{attribute 'qualified_only'}
VAR_GLOBAL
//************************HW-IO******************************************
	NDI:STR_NDI;	
	NDO:STR_NDO;
	AI:STR_AI;
	AO:STR_AO;
	
	//POWER
	TURBO_PUMP_POWER_ON :BOOL;
	PENDULUM_VALVE_HEATER_POWER_ON:BOOL;
	LID_HEATER_POWER_ON:BOOL;
	CHAMBER_HEATER_POWER_ON:BOOL;
	IGS_HEATER_POWER_ON:BOOL;
	TAPE_HEATER_POWER_ON:BOOL;
	FORELINE_HEATER_POWER_ON:BOOL;
	GATE_VALVE_HEATER_POWER_ON:BOOL;
	
	//HEATER	
	LID_HEATER_AUTO_TUNE_EN				:ARRAY[1..10] OF BOOL;
	CHAMBER_HEATER_AUTO_TUNE_EN			:ARRAY[1..10] OF BOOL;
	PEN_VALVE_HEATER_AUTO_TUNE_EN		:BOOL;
	GATE_VALVE_HEATER_AUTO_TUNE_EN		:BOOL;
	IGS_HEATER_AUTO_TUNE_EN				:ARRAY[1..10] OF BOOL;
	TAPE_HEATER_AUTO_TUNE_EN			:ARRAY[1..10] OF BOOL;
	FORELINE_HEATER_AUTO_TUNE_EN		:ARRAY[1..20] OF BOOL;
	STAGE_HEATER_AUTO_TUNE_EN			:ARRAY[1..10] OF BOOL;
	
	LID_HEATER_AUTO_TUNE_OUTPUT			:ARRAY[1..10] OF REAL;
	CHAMBER_HEATER_AUTO_TUNE_OUTPUT		:ARRAY[1..10] OF REAL;
	PEN_VALVE_HEATER_AUTO_TUNE_OUTPUT	:REAL;
	GATE_VALVE_HEATER_AUTO_TUNE_OUTPUT	:REAL;
	IGS_HEATER_AUTO_TUNE_OUTPUT			:ARRAY[1..10] OF REAL;
	TAPE_HEATER_AUTO_TUNE_OUTPUT		:ARRAY[1..10] OF REAL;
	FORELINE_HEATER_AUTO_TUNE_OUTPUT	:ARRAY[1..20] OF REAL;
	STAGE_HEATER_AUTO_TUNE_OUTPUT		:ARRAY[1..10] OF REAL;
	
	LID_HEATER_SSR_ON					:ARRAY[1..10] OF BOOL;
	CHAMBER_HEATER_SSR_ON				:ARRAY[1..10] OF BOOL;
	PEN_VALVE_HEATER_SSR_ON				:BOOL;
	GATE_VALVE_SSR_ON					:BOOL;
	IGS_HEATER_SSR_ON					:ARRAY[1..10] OF BOOL;
	TAPE_HEATER_SSR_ON					:ARRAY[1..10] OF BOOL;
	FORELINE_HEATER_SSR_ON				:ARRAY[1..20] OF BOOL;
	STAGE_HEATER_SCR_OUTPUT				:ARRAY[1..10] OF REAL;
	
//INTERLOCK
	ALARM_OCC:BOOL;
	WARNING_OCC:BOOL;
	
//UI-Config
	PMConfig:ConfigPM;
	
	MFCVerification:ConfigMfcVer;
	
	Chiller:ConfigChiller;	
	InnerChiller:ConfigChiller;
	OuterChiller:ConfigChiller;
	TopChiller:ConfigChiller;
	
	DryPump:ConfigDryPump;
	
	Mfcgas1					:ConfigMfcGas;
	Mfcgas2					:ConfigMfcGas;
	Mfcgas3					:ConfigMfcGas;
	Mfcgas4					:ConfigMfcGas;
	Mfcgas5					:ConfigMfcGas;
	Mfcgas6					:ConfigMfcGas;
	Mfcgas7					:ConfigMfcGas;
	Mfcgas8					:ConfigMfcGas;
	Mfcgas9					:ConfigMfcGas;
	Mfcgas10				:ConfigMfcGas;
	Mfcgas11				:ConfigMfcGas;
	Mfcgas12				:ConfigMfcGas;	
	MfcN2					:ConfigMfcGas;
	MfcHe					:ConfigMfcGas; 
	
	Pump:ConfigPump;
	
	Purge:ConfigPurge;
	
	PendulumHeater:ConfigHeater;
	LidHeater:ConfigHeater;
	ChamberHeater:ConfigHeater;
	IGSHeater:ConfigHeater;
	TapeHeater:ConfigHeater;
	ForelineHeater:ConfigHeater;
	STAGE:ConfigHeater;
	
	ElectrostaticVoltageSource:ConfigElectrostaticVoltageSource;
	
	TurboPump:ConfigTurboPump;
	
	PendulumValve:ConfigPendulumValve;
	
	IdleClean:ConfigIdleClean;
	
	EPD:ConfigEPD;
	
	HighTemperatureChiller:ConfigHighTempChiller;
		
	
//UI-RECIPE
	Step_Num:INT;
	SetpArray:ARRAY[1..100] OF RecipeEachStep;
	
//INTERLOCK
	TurboN2PurgePressure:INT;	//PS103	
	
	Process_Start:BOOL;
	Process_Stop:BOOL;
END_VAR
